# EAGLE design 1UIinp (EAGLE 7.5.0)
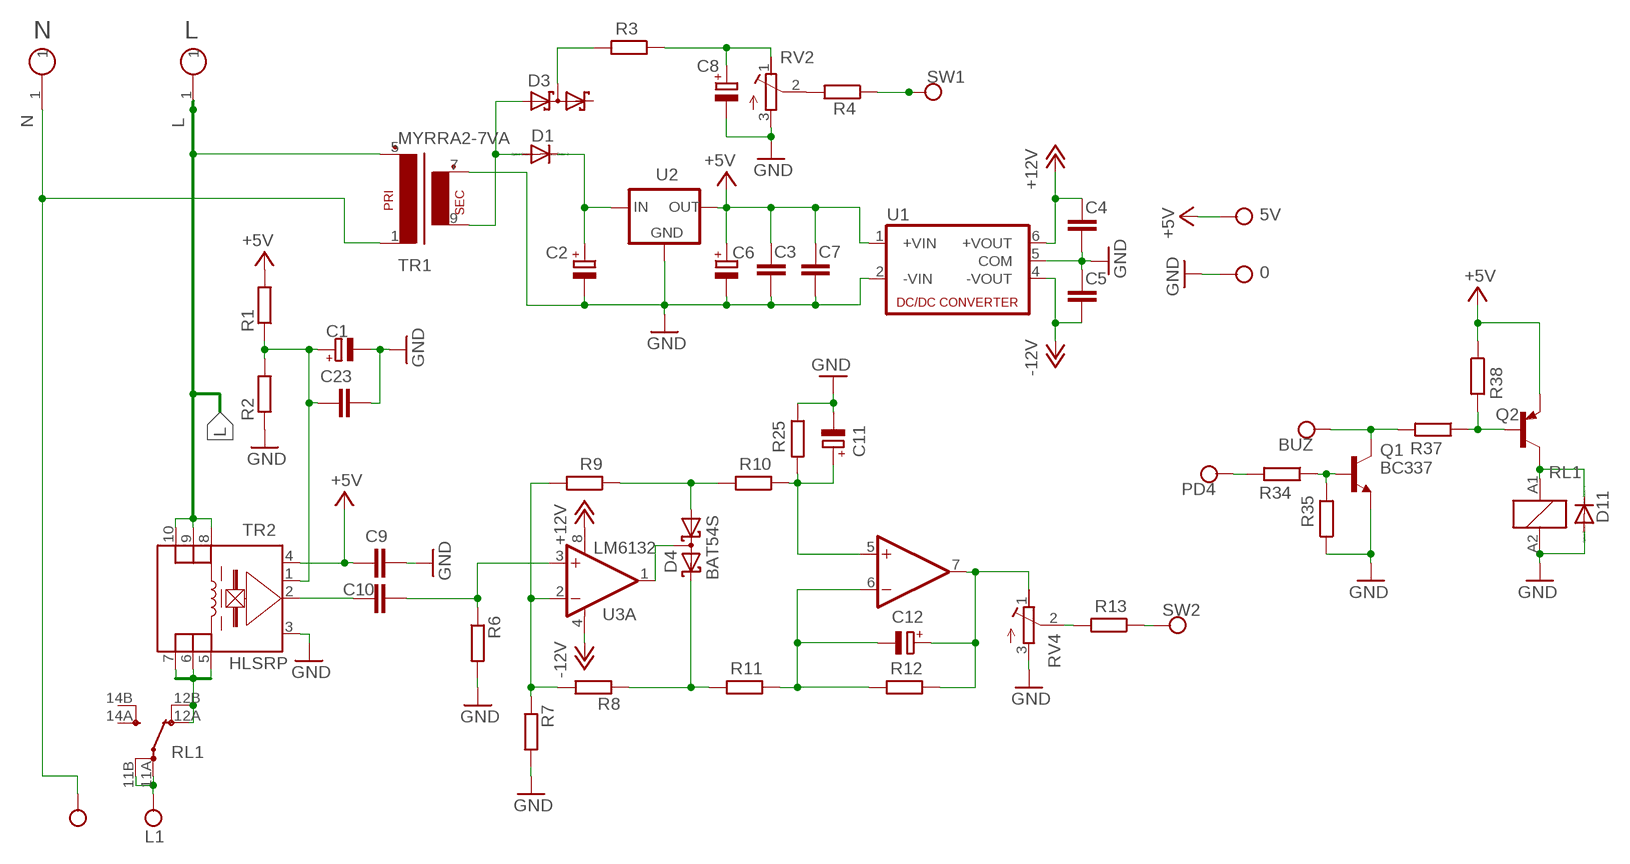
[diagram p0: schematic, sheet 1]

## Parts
0  CONNWIRE  [CONNWIRE]
5V  CONNWIRE  [CONNWIRE]
BUZ  CONNWIRE  [CONNWIRE]
C1  CPOL-EUE2-5  [E2-5]
C2  CPOL-EUE5-8.5  [E5-8,5]
C3  C-EUC1206  [C1206]
C4  C-EUC1206  [C1206]
C5  C-EUC1206  [C1206]
C6  CPOL-EUE2-5  [E2-5]
C7  C-EUC1206  [C1206]
C8  CPOL-EUE3.5-8  [E3,5-8]
C9  C-EUC1206  [C1206]
C10  C-EUC1206  [C1206]
C11  CPOL-EUE2-5  [E2-5]
C12  CPOL-EUE2-5  [E2-5]
C23  C-EUC1206  [C1206]
D1  1N4004  [DO41-10]
D3  BAT54S  [SOT23]
D4  BAT54S  [SOT23]
D11  1N4004  [DO41-10]
L  CONNHOLE  [CONNHOLE4]
L1  CONNWIRE2MM  [CONNVIRE2MM]
N  CONNHOLE  [CONNHOLE4]
N1  CONNWIRE  [CONNWIRE]
PD4  CONNWIRE  [CONNWIRE]
Q1  BC337  [TO92]
Q2  -PNP-TO126  [TO126]
R1  R-EU_0204/7  [0204/7]
R2  R-EU_0204/7  [0204/7]
R3  R-EU_0204/7  [0204/7]
R4  R-EU_0204/7  [0204/7]
R6  R-EU_0204/7  [0204/7]
R7  R-EU_0204/7  [0204/7]
R8  R-EU_0204/7  [0204/7]
R9  R-EU_0204/7  [0204/7]
R10  R-EU_0204/7  [0204/7]
R11  R-EU_0204/7  [0204/7]
R12  R-EU_0204/7  [0204/7]
R13  R-EU_0204/7  [0204/7]
R25  R-EU_0204/7  [0204/7]
R34  R-EU_0204/7  [0204/7]
R35  R-EU_0204/7  [0204/7]
R37  R-EU_0204/7  [0204/7]
R38  R-EU_0204/7  [0204/7]
RL1  RZ03-1A4-D005  RTH14012  [RT-C/O16A5]
RV2  R-TRIMM-3386-F  [R-TRIMM-3386F]
RV4  R-TRIMM-3386-F  [R-TRIMM-3386F]
SW1  CONNWIRE  [CONNWIRE]
SW2  CONNWIRE  [CONNWIRE]
TR1  MYRRA2-7VA  [MYRRA2-7]
TR2  HLSRP  [HLRSXPSP]
U1  NMA  [NMA]
U2  78XXL  [78XXL]
U3  LM6132  OPA2134P  [DIL08]

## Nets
+5V: 5V.P$1 C3.1 C6.+ C7.1 C9.1 Q2.1(E) R1.2 R38.1 TR2.4(V+) U1.1(+VIN) U2.OUT
+12V: C4.1 U1.6(+VOUT) U3.8(A:V+)
-12V: C5.2 U1.4(-VOUT) U3.4(A:V-)
GND: 0.P$1 C1.- C2.- C3.2 C4.2 C5.1 C6.- C7.2 C8.- C9.2 C11.- C23.2 D11.A Q1.1(E) R2.1 R6.2 R7.2 R25.1 R35.1 RL1.A2 RV2.3(E) RV4.3(E) TR1.7(S3) TR2.3 U1.2(-VIN) U1.5(COM) U2.GND
L: L.1 TR1.5(P2) TR2.8(1I+) TR2.9(2I+) TR2.10(3I+)
N$1: C10.1 TR2.2
N$3: D3.3(C1A2) R3.2
N$4: R7.1 R8.2 R9.2 U3.2(A:-IN)
N$5: C10.2 R6.1 U3.3(A:+IN)
N$6: RL1.12A(2:OA) RL1.12B(2:OB) TR2.5(4I-) TR2.6(5I-) TR2.7(6I-)
N$8: D4.2(C2) R8.1 R11.2
N$10: C11.+ R10.1 R25.2 U3.5(B:+IN)
N$11: C12.- R11.1 R12.2 U3.6(B:-IN)
N$12: R4.2 RV2.2(S)
N$13: R4.1 SW1.P$1
N$14: R13.2 RV4.2(S)
N$24: D4.3(C1A2) U3.1(A:OUT)
N$29: D1.A D3.1(A1) TR1.9(S4)
N$31: D4.1(A1) R9.1 R10.2
N$33: C12.+ R12.1 RV4.1(A) U3.7(B:OUT)
N$37: C2.+ D1.C U2.IN
N$40: C8.+ R3.1 RV2.1(A)
N$44: R13.1 SW2.P$1
N$48: Q1.2(B) R34.1 R35.2
N$49: BUZ.P$1 Q1.3(C) R37.2
N$50: Q2.3(B) R37.1 R38.2
N$51: PD4.P$1 R34.2
N$63: D11.C Q2.2(C) RL1.A1
N$66: L1.1 RL1.11A(2:PA) RL1.11B(2:PB)
N$70: N1.P$1 N.1 TR1.1
UREF: C1.+ C23.1 R1.1 R2.2 TR2.1
Unconnected: D3.2(C2) RL1.14A(2:SA) RL1.14B(2:SB)

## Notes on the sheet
- N | L

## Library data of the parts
0 5V BUZ N1 PD4 SW1 SW2 = connholes:CONNWIRE
C1 C2 C6 C8 C11 C12 = rcl:CPOL-EU: POLARIZED CAPACITOR, European symbol
C3-C5 C7 C9 C10 C23 = rcl:C-EU: CAPACITOR, European symbol
D1 D11 = diode:1N4004: DIODE
D3 D4 = diode:BAT54S: Schottky Diodes Pin connection corrected 2011-05-04 Source: Fairchild .. BAT54.pdf
L N = connholes:CONNHOLE
L1 = connholes:CONNWIRE2MM
Q1 = transistor:BC337: NPN TRANSISTOR
Q2 = transistor:*-PNP-: PNP Transistror
R1-R4 R6-R13 R25 R34 R35 R37 R38 = rcl:R-EU_: RESISTOR, European symbol
RL1 = relay:RTH14*: Power PCB Relay 105°C 16A SCHRACK 1 pole 16 A, high-temperature version Source: http://www.schrack.com/.. 5831.pdf; MPN: RTH14012; OC_FARNELL: 1629018; OC_NEWARK: 03P2408
RV2 RV4 = rcl:R-TRIMM-3386-F
TR1 = trafo:MYRRA2-7VA
TR2 = lem:HLSRP
U1 = dc-dc-converter:NMA: DC-DC CONVERTER; MF: C & D TECHNOLOGIES, INC; MPN: NMA0515SC; OC_FARNELL: 1021434; OC_NEWARK: 61K3064
U2 = v-reg:78XXL: VOLTAGE REGULATOR
U3 = burr-brown:OPA2134: Operational Amplifier; MF: TEXAS INSTRUMENTS; MPN: OPA2134PA; OC_FARNELL: 1097574; OC_NEWARK: 74K3897

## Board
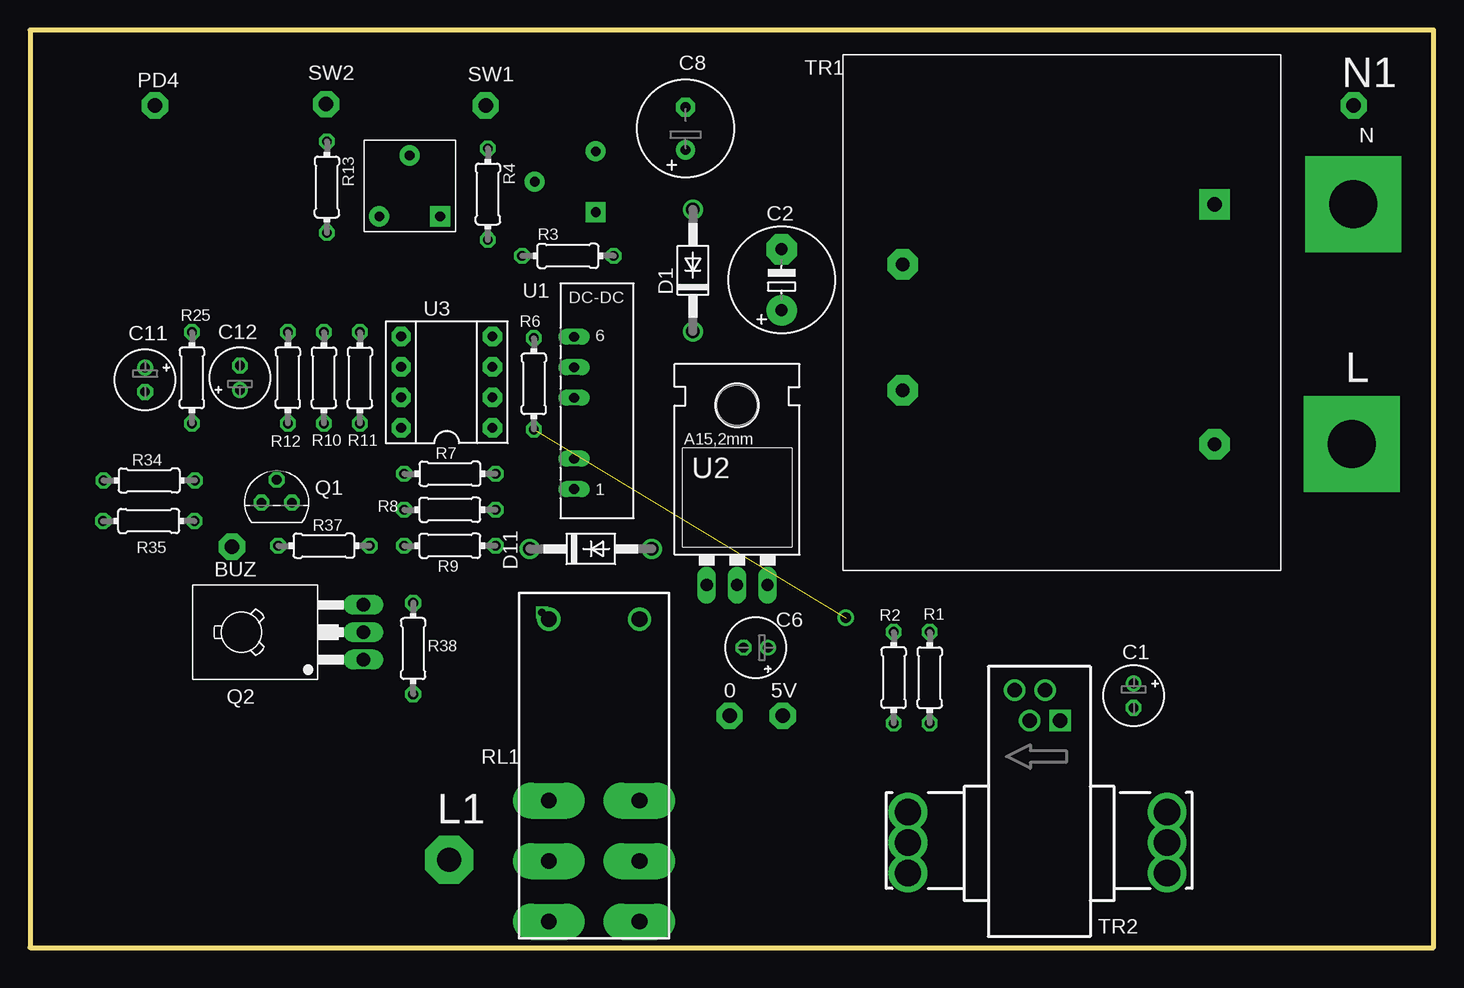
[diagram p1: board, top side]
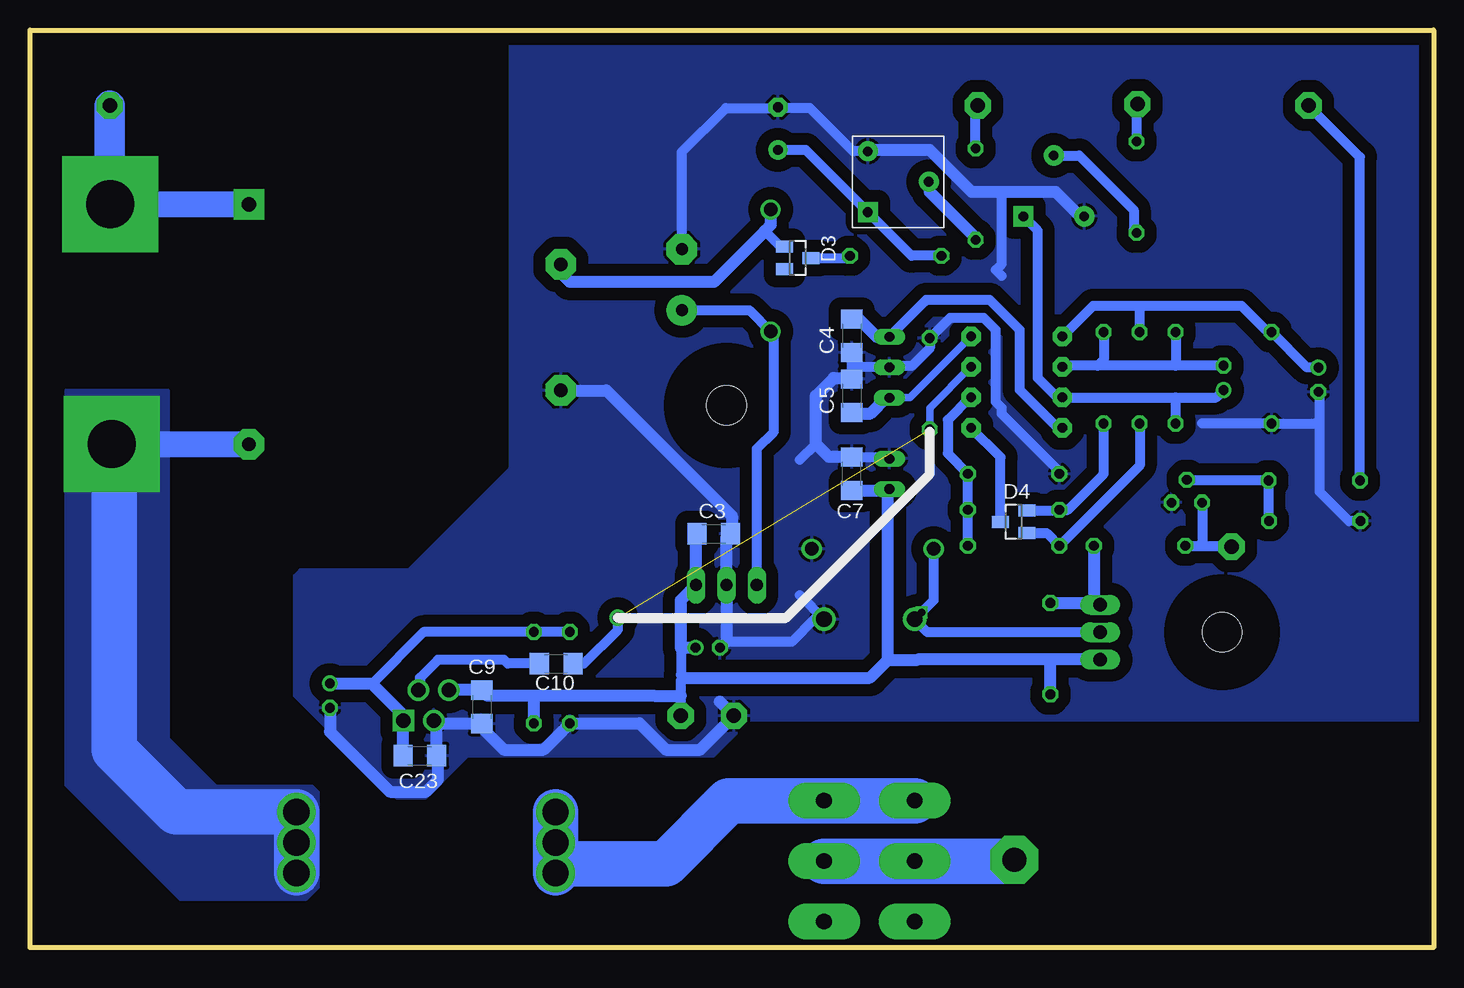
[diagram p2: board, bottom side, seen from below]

Size 117 x 76.5 mm. Coordinates in mm from the lower left corner, seen from the top.
Outline: 0,0 117,0 117,76.5 0,76.5 0,0
Copper layers (1*16): Top 0.035mm / dielectric 1.5mm / Bottom 0.035mm
Design rules "default": minimum track width 10mil, minimum drill 24mil, track to track 8mil, track to pad 8mil, pad to pad 8mil, via to via 8mil, smd to smd 8mil, copper to edge 40mil, drill to drill 8mil, minimum pad ring 10mil, minimum via ring 8mil, stop-mask expansion 4mil, vias tented up to drill 0mil, thermal gap 10mil

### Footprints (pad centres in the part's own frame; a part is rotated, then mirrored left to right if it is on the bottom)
CONNWIRE = drill 1.2 pad 2.184 octagon: P$1 0,0
E2-5 = drill 0.813 pad 1.27: + -1.016,0 | drill 0.813 pad 1.27 octagon: - 1.016,0
E5-8,5 = drill 1.016 pad 2.54: + -2.54,0 | drill 1.016 pad 2.54 octagon: - 2.54,0
C1206 = smd 1.6 x 1.8: 1 -1.4,0; 2 1.4,0
E3,5-8 = drill 0.813 pad 1.6: + -1.778,0 | drill 0.813 pad 1.6 octagon: - 1.778,0
DO41-10 = drill 1.118: A 5.08,0; C -5.08,0
SOT23 = smd 1 x 1.4: 1 -0.95,-1.1; 2 0.95,-1.1; 3 0,1.1
CONNHOLE4 = drill 4 pad 8 square: 1 0,0
CONNVIRE2MM = drill 2 pad 4 octagon: 1 0,0
TO92 = drill 0.813 octagon: 1 1.27,0; 2 0,1.905; 3 -1.27,0
TO126 = drill 1.118 long: 1 -2.286,-5.08; 2 0,-5.08; 3 2.286,-5.08 | hole 3.302: 0,5.08
0204/7 = drill 0.813 octagon: 1 -3.81,0; 2 3.81,0
RT-C/O16A5 = drill 1.3 pad 3 long: 11A 7.56,3.78; 11B 7.56,-3.78; 12A 2.52,3.78; 12B 2.52,-3.78; 14A 12.6,3.78; 14B 12.6,-3.78 | drill 1.3: A1 -12.6,-3.78; A2 -12.6,3.78
R-TRIMM-3386F = drill 0.8 pad 1.676 square: 1 0,0 | drill 0.8 pad 1.676: 2 5.08,2.54; 3 0,5.08
MYRRA2-7 = drill 1.2 pad 2.54 square: 1 0,0 | drill 1.1 pad 2.54 octagon: 5 20,0; 7 15.5,-26; 9 5,-26
HLRSXPSP = drill 1.2 square: 1 0,0 | drill 1.2: 2 1.27,-2.54; 3 2.54,0; 4 3.81,-2.54 | drill 2.2 pad 3.1: 5 12.7,7.62; 6 12.7,10.16; 7 12.7,12.7; 8 -8.89,12.7; 9 -8.89,10.16; 10 -8.89,7.62
NMA = drill 0.813 long: 1 0,6.35; 2 0,3.81; 4 0,-1.27; 5 0,-3.81; 6 0,-6.35
78XXL = drill 1.016 long: GND 0,-3.81; IN -2.54,-3.81; OUT 2.54,-3.81 | hole 3.302: 0,11.176
DIL08 = drill 0.813 pad 1.6 octagon: 1 -3.81,-3.81; 2 -1.27,-3.81; 3 1.27,-3.81; 4 3.81,-3.81; 5 3.81,3.81; 6 1.27,3.81; 7 -1.27,3.81; 8 -3.81,3.81

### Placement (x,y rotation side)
0  58.32,19.32 0 top
5V  62.75,19.32 0 top
BUZ  16.83,33.42 0 top
C1  92,21 270 top
C2  62.65,55.68 90 top
C3  60,34.5 0 bottom
C4  48.5,51 270 bottom
C5  48.5,46 270 bottom
C6  60.5,25 180 top
C7  48.5,39.5 90 bottom
C8  54.65,68.28 90 top
C9  79.33,20.06 270 bottom
C10  73.14,23.67 0 bottom
C11  9.59,47.34 270 top
C12  17.5,47.5 90 top
C23  84.5,16 0 bottom
D1  55.26,56.45 90 top
D3  53,57.5 270 bottom
D4  35,35.5 90 bottom
D11  46.75,33.24 0 top
L  110.19,41.99 0 top
L1  34.94,7.31 0 top
N  110.3,61.99 0 top
N1  110.35,70.2 0 top
PD4  10.42,70.2 0 top
Q1  20.56,37.09 0 top
Q2  22.7,26.29 90 top
R1  75,22.5 270 top
R2  72,22.5 90 top
R3  44.84,57.67 0 top
R4  38.17,62.82 270 top
R6  42,47 90 top
R7  35,39.5 180 top
R8  35,36.5 0 top
R9  35,33.5 0 top
R10  24.5,47.5 270 top
R11  27.5,47.5 270 top
R12  21.5,47.5 90 top
R13  24.75,63.4 270 top
R25  13.5,47.5 90 top
R34  9.94,38.94 180 top
R35  9.9,35.56 0 top
R37  24.5,33.5 180 top
R38  31.94,24.92 90 top
RL1  47.03,14.76 270 top
RV2  47.15,61.31 0 bottom
RV4  34.19,60.96 90 top
SW1  37.99,70.2 0 top
SW2  24.68,70.32 0 top
TR1  98.75,61.95 270 top
TR2  85.89,18.92 180 top
U1  45.36,44.57 180 top
U2  58.95,34.03 0 top
U3  34.74,47.14 90 top

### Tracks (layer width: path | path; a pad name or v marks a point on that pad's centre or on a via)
+5V
  Bottom 0.813: R38.1 31.94,21.44 | 62.75,25 62.75,22.75 62.5,22.5 62.75,22.25 62.75,21 5V.P$1
  Bottom 1.016: TR2.4 C9.1 78.87,21 75,21 | 75,21 65,21 62.75,21 | C6.+ 62.75,25 62.75,28.96 U2.OUT 61.49,34.41 C3.1 | 45.5,24 45.5,38.08 U1.1 45.48,38.1 C7.1 | R1.2 75,21 | Q2.1 32,24 | 32,24 43,24 43.01,24 45.5,24 | 31.94,21.44 31.94,23.94 32,24 | 62.5,22.5 47,22.5 45.5,24
+12V
  Bottom 0.813: U3.8 31.33,43.33 34.5,46.5 34.5,51.5 37,54 42.28,54 42.39,53.89 U1.6
  Bottom 1.016: U1.6 46.42,50.92 48,52.5 48.4,52.5 C4.1
-12V
  Bottom 0.61: U1.4 43.66,45.84 U3.4
  Bottom 1.016: U1.4 45.66,45.84 47,44.5 48.4,44.5 C5.2
GND
  Bottom 0.813: 58.95,25.53 58.92,25.5 53.5,25.5 51.64,27.36 RL1.A2 52.83,29.38 | C2.- 62.65,66.35 59,70 54.71,70 C8.- 54.59,70 52,70 48.39,66.39 RV2.3 | C5.1 48.5,48.5 | 48.5,48.5 C4.2 | 48.5,48.5 48.38,48.38 U1.5 45.24,48.5 43.5,48.5 42,50 R6.2 40.31,52.5 37.5,52.5 36.5,51.5 36.5,45.5 36,45 36,44.5 31.19,39.69 R7.2 | 52.83,40.67 51.5,42 | 36,56 36.5,56.5 36,57 36,63 | C7.2 45.5,40.9 U1.2 | 19.31,43.69 R25.1 9.81,43.69 9.5,44 | R35.1 7.06,35.56 9.5,38 9.5,44 | 9.5,44 9.5,46.23 C11.-
  Bottom 1.016: C1.- 92,18 87,13 84,13 83,14 83,15.9 C23.2 83.1,18.67 TR2.3 83.09,18.66 C9.2 79.33,18.33 77.5,16.5 74.19,16.5 R2.1 66.19,18.69 64,16.5 61.14,16.5 0.P$1 59.48,20.48 | C6.- 58.95,25.53 U2.GND 58.95,34.15 C3.2 58.5,34.6 58.5,36 68.95,46.45 TR1.7 | RV4.3 29.46,60.96 31.5,63 36,63 38.5,63 42,66.5 47.04,66.5 RV2.3 | R6.2 42,51 | C7.2 50.4,40.9 51.5,42 51.5,46 50,47.5 48.6,47.5 C5.1
  pour Bottom (isolate 1.016): 1.5,75.5 77,75.5 77,40 85.5,31.5 94.5,31.5 95,31 95,21 86.5,12.5 84,12.5 80.5,16 60,16 57,19 1,19 1,75.5
L
  Bottom 2.184: L.1 98.79,41.99 TR1.5
  Bottom 3.81: TR2.8 TR2.9 TR2.10 104.8,11.3 110,16.5 110,41.8 L.1
  pour Bottom (no thermals): 105.5,46.5 105.5,17.5 101.5,13.5 93.5,13.5 93,13 93,5 94,4 104.5,4 114,13.5 114,46.5
N$1
  Bottom 0.813: C10.1 77.17,23.67 77.5,24 83,24 84.5,22.5 84.5,21.58 TR2.2
N$3
  Bottom 0.813: D3.3 48.82,57.5 R3.2
N$4
  Bottom 0.813: R9.2 R8.2 R7.1 40.5,41.19 40.5,44 38.63,45.87 U3.2
N$5  (via drill 0.9)  (1 unrouted)
  Bottom 0.61: U3.3 38.59,48.41 42,45 R6.1
  Bottom 0.813: C10.2 70.83,23.67 68,26.5 v68,27.5
N$6
  Bottom 3.81: TR2.5 TR2.6 TR2.7 72.41,7 64,7 58.76,12.24 RL1.12A RL1.12B
N$8
  Bottom 0.813: D4.2 31.24,36.45 R8.1 30.5,36.5 27.5,39.5 R11.2
N$10
  Bottom 0.813: C11.+ 10.55,48.36 R25.2 13.81,51.31 16,53.5 24.5,53.5 | 24.5,53.5 28.38,53.5 U3.5 | R10.1 24.5,53.5
N$11
  Bottom 0.813: C12.- 21.5,48.52 | 21.5,48.52 28,48.52 | 28,48.52 30.82,48.52 U3.6 | R12.2 21.5,48.52 | R11.1 27.5,49.02 28,48.52
N$12
  Bottom 1.016: R4.2 38.17,59.17 42,63 42,63.78 RV2.2
N$13
  Bottom 0.813: R4.1 38.17,70.02 SW1.P$1
N$14
  Bottom 0.813: RV4.2 29.54,66.04 25,61.5 25,59.84 R13.2
N$24
  Bottom 0.813: D4.3 36.1,40.88 U3.1
N$29
  Bottom 0.813: D3.1 54.45,58.45 55.75,59.75
  Bottom 1.016: D1.A 55.26,60.24 55.75,59.75 60,55.5 72,55.5 73,56.5 73,56.7 TR1.9
N$31
  Bottom 0.813: R10.2 24.5,40.19 R9.1 32.24,34.55 D4.1
N$33
  Bottom 0.813: 21.5,45.87 U3.7 31.37,45.87 33,47.5 33,59.77 RV4.1 34,60.77 | 21.5,45.87 18.11,45.87 C12.+ | R12.1 21.5,45.87
N$37
  Bottom 0.813: C2.+ 57.03,53.14 D1.C 55,51.11 55,43 56.41,41.59 U2.IN
N$40
  Bottom 0.813: R3.1 43.51,57.67 RV2.1 52.34,66.5 C8.+
N$44
  Bottom 0.813: R13.1 24.75,70.25 SW2.P$1
N$48
  Bottom 0.813: Q1.2 20.5,38.94 R34.1 13.71,38.9 R35.2
N$49
  Bottom 0.813: R37.2 19,33.5 | 19,33.5 16.91,33.5 BUZ.P$1 | Q1.3 19.29,33.79 19,33.5
N$50
  Bottom 1.016: R37.1 28.31,29.11 Q2.3 27.93,28.73 R38.2
N$51
  Bottom 0.813: R34.2 6.13,65.91 PD4.P$1
N$63  (via drill 0.6)
  Bottom 0.813: v42.67,27.94 RL1.A1 | Q2.2 42.18,26.29 RL1.A1 | D11.C 41.67,28.94 RL1.A1
N$66
  Bottom 3.81: RL1.11A RL1.11B 35.05,7.2 L1.1
N$70
  Bottom 2.184: N.1 98.79,61.99 TR1.1
  Bottom 2.54: N1.P$1 110.35,62.04 N.1
UREF
  Bottom 0.813: 88.5,22 84.19,26.31 R1.1 R2.2
  Bottom 1.016: C23.1 TR2.1 | TR2.1 | TR2.1 85.9,19.4 88.5,22 91.98,22 C1.+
